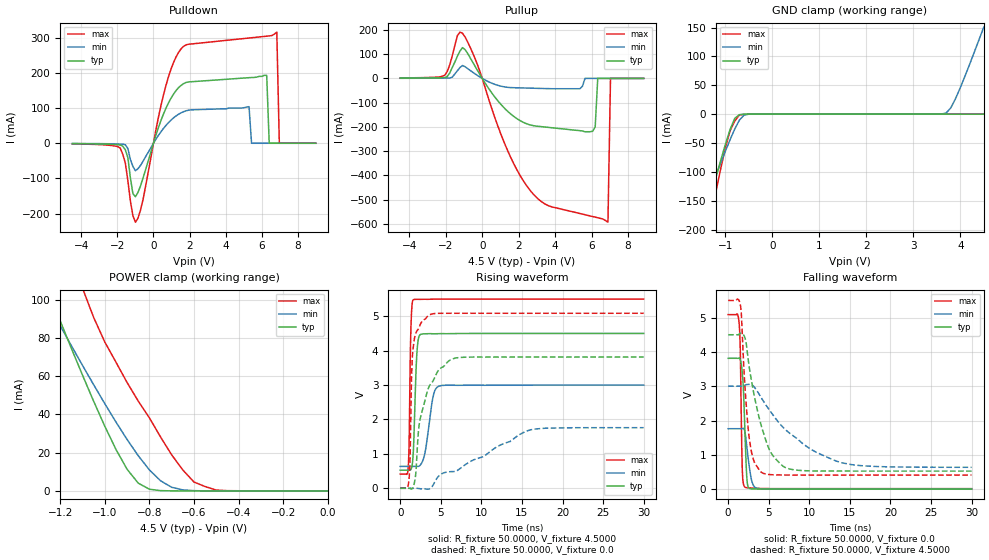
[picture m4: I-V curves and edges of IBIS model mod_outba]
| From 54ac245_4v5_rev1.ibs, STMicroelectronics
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|   Model mod_outba
[Model]   mod_outba
Model_type 3-state
Enable   Active-Low
Vmeas   =  2.25V
Rref   =  500
Cref   =  50pF
C_comp   3.517pF   NA   NA
[Temperature Range]   25.0000   0.1250k   -55.0000
[Voltage Range]   4.5000V   3.0000V   5.5000V
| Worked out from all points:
|   slope of the pulldown table from 0 to 0.675 V, typ, clamps not added: 6.92 ohm
|   slope of the pullup table from 0 to 0.675 V, typ, clamps not added: 8.98 ohm
|   GND clamp passes 1 mA (typ) near -0.70 V on its own axis
|   POWER clamp passes 1 mA (typ) near -0.80 V on its own axis
|   rising waveform, R_fixture 50.0000, V_fixture 4.5000: 20-80 % time 342ps typ, 830ps min, 197ps max; typ from 0.527 V to 4.5 V
|   rising waveform, R_fixture 50.0000, V_fixture 0.0: 20-80 % time 1.82ns typ, 9.08ns min, 364ps max; typ from 0 V to 3.81 V
|   falling waveform, R_fixture 50.0000, V_fixture 0.0: 20-80 % time 360ps typ, 587ps min, 204ps max; typ from 3.81 V to 0 V
|   falling waveform, R_fixture 50.0000, V_fixture 4.5000: 20-80 % time 2.28ns typ, 6.15ns min, 882ps max; typ from 4.5 V to 0.527 V
[Pulldown]
|Voltage   I(typ)   I(min)   I(max)
-4.5V     -1.1mA     -680uA     -2mA
-1.84V    -4.97mA    -2.36mA    -13.95mA
-1V       -152mA     -78mA      -224.4mA
680mV     98.1mA     49.9mA     161.9mA
1.52V     164.1mA    86.21mA    267.6mA
5.3V      186.4mA    104mA      299.2mA
5.44V     186.9mA    0A         299.9mA
6.28V     193mA      0A         304.4mA
6.42V     0A         0A         305.1mA
6.84V     0A         0A         316mA
6.98V     0A         0A         0A
9V        0A         0A         0A
[Pullup]
|Voltage   I(typ)   I(min)   I(max)
-4.5V     1mA        440uA      1.9mA
-2.06V    3.34mA     1.31mA     12.89mA
-1.36V    92.46mA    32mA       177mA
-1.08V    127mA      53mA       186mA
1.02V     -106.7mA   -31.88mA   -229.1mA
2.56V     -190.3mA   -40.04mA   -455.1mA
6.06V     -218mA     0A         -569.7mA
6.2V      -200mA     0A         -572.2mA
6.34V     0A         0A         -574.7mA
6.9V      0A         0A         -593mA
7.04V     0A         0A         0A
8.86V     0A         0A         0A
[GND_clamp]
|Voltage   I(typ)   I(min)   I(max)
-4.5V     -1.129A    -845.6mA   -1.584A
-1.7V     -259.6mA   -215.1mA   -344.2mA
-1.6V     -229.1mA   -193mA     -301.2mA
-1.5V     -198.8mA   -171.1mA   -258.4mA
-1.4V     -168.7mA   -149.2mA   -216.2mA
-1.3V     -138.8mA   -127.6mA   -174.5mA
-900mV    -26.79mA   -44.34mA   -28.98mA
-700mV    -976uA     -10.21mA   -1.6mA
-500mV    -12uA      -127.7uA   -211uA
3.7V      89.43pA    1.897mA    5.074pA
3.9V      94.16pA    26.87mA    5.078pA
4.5V      112.8pA    150.7mA    5.087pA
[POWER_clamp]
|Voltage   I(typ)   I(min)   I(max)
-4.5V     1.107A     824.5mA    1.575A
-1.3V     118.1mA    107.6mA    178.8mA
-1.25V    103.4mA    96.95mA    159.5mA
-1.1V     60.56mA    65.66mA    106mA
-950mV    21.72mA    36.02mA    67.3mA
-900mV    11.32mA    26.87mA    56.66mA
-850mV    4.056mA    18.4mA     46.92mA
-750mV    159.2uA    5.291mA    28.18mA
-700mV    29.54uA    1.897mA    18.82mA
-600mV    1.685uA    128.9uA    4.628mA
-500mV    160.8nA    7.103uA    429uA
0V        112.8pA    2.644nA    186.4pA
[Ramp]
| variable   typ   min   max
dV/dt_r  2.2880/1.8154n   1.0574/8.9233n   3.0429/0.3776n
dV/dt_f  2.3845/2.2675n   1.4184/6.1217n   3.0523/0.9248n
R_load = 50.0000
[Rising Waveform]
R_fixture= 50.0000
V_fixture= 4.5000
V_fixture_min= 3.0000
V_fixture_max= 5.5000
|time   V(typ)   V(min)   V(max)
0s        526.6mV    636.6mV    411.9mV
960ps     526.6mV    636.6mV    542.3mV
1.08ns    527.5mV    636.6mV    1.16V
1.32ns    552mV      636.6mV    4.694V
1.62ns    1.089V     636.6mV    5.481V
2.04ns    3.881V     637mV      5.492V
2.52ns    4.473V     690.2mV    5.491V
4.08ns    4.49V      2.695V     5.496V
4.8ns     4.493V     2.97V      5.499V
30ns      4.5V       3V         5.499V
[Rising Waveform]
R_fixture= 50.0000
V_fixture= 0.0
V_fixture_min= 0.0
V_fixture_max= 0.0
|time   V(typ)   V(min)   V(max)
0s        187pV      296.7pV    15.22mV
1.11ns    1.45mV     323.3nV    333.9mV
1.23ns    -8.547mV   992.3nV    1.042V
1.41ns    -20.13mV   2.744uV    3.36V
1.74ns    152.4mV    -67.27uV   4.338V
2.34ns    1.858V     -9.879mV   4.676V
3.48ns    2.917V     -24.73mV   5.02V
6.72ns    3.78V      487.1mV    5.087V
16.08ns   3.814V     1.7V       5.087V
30ns      3.814V     1.762V     5.087V
[Falling Waveform]
R_fixture= 50.0000
V_fixture= 0.0
V_fixture_min= 0.0
V_fixture_max= 0.0
|time   V(typ)   V(min)   V(max)
0s        3.814V     1.762V     5.087V
1.32ns    3.823V     1.762V     4.916V
1.5ns     3.77V      1.761V     4.002V
1.74ns    3.4V       1.765V     573.6mV
1.86ns    3.017V     1.774V     178.6mV
2.07ns    1.667V     1.661V     60.01mV
2.34ns    217.8mV    1.155V     42.01mV
2.7ns     14.14mV    502.6mV    37.53mV
3.96ns    2.684mV    13.02mV    20.64mV
30ns      -45.59nV   4.836uV    15.22mV
[Falling Waveform]
R_fixture= 50.0000
V_fixture= 4.5000
V_fixture_min= 3.0000
V_fixture_max= 5.5000
|time   V(typ)   V(min)   V(max)
0s        4.5V       3V         5.499V
1.47ns    4.539V     3V         5.41V
1.62ns    4.545V     2.999V     5.125V
2.13ns    4.363V     3.037V     2.777V
2.61ns    3.538V     3.052V     1.462V
4.11ns    1.825V     2.654V     489.4mV
5.25ns    1.076V     2.254V     422.6mV
6.99ns    637.9mV    1.749V     412.6mV
13.32ns   527.1mV    819mV      411.9mV
30ns      526.6mV    636.9mV    411.9mV
